|   IBIS model for TI xxx DSP
[IBIS Ver]   5.1
[Disclaimer]   Please be aware that in the absence of a written agreement
|   Texas Instruments(TI) assumes no liability for:
|   (1) The accuracy of the IBIS models provided to your company,
|   however, the IBIS model is compliant to industry standard
|   IQ Level 2a.  Refer to IBIS Quality Section below for
|   for full details.
|   (2) The proper functioning of these Models in your design
|   or for any resulting applications
|   (3) Infringement of patents, copyrights or intellectual
|   property rights resulting from your use of these
|   models.
|   TI provides IBIS Models as a service to our customers and
|   therefore reserves the right to limit distribution of the
|   Models.  The information is subject to change without notice.
[File Name]  sprm806c.ibs
[File Rev]   0.4
|   -Initial version
|   - Fixed component name
|   - Removed unsupported drive strengths for LVCMOS and SDIO models
|   - Removed unsupported drive strengths for LVDS, IIC and eMMC buffer models
[Date]   20 Oct 2023
[Source]   Texas Instruments Incorporated
[Copyright]   Property of Texas Instruments Incorporated.
|   Unauthorized reproduction and/or distribution is strictly.
|   prohibited.
|   This product is protected under copyright law and trade
|   secret law as an unpublished work.
|   Created 2012,(C) Copyright 1999-2012,
|   Texas Instruments Incorporated., All Rights Reserved.
|   These commodities are under the U.S. Government
|   distribution license control. As such,they are not to be
|   re-exported without the prior approval of the U.S.
|   Department of Commerce.
[Notes]
   This file does not include AMI models for SerDes based links.
   For SerDes simulations use Texas Instruments IBIS AMI models
   Some IV curves contain Non monotonic data points.
|   Revision History
|   GERNERAL COMMENT: All IBIS Quality Notes below reflect latest release
|   and version of IBIS File
|   File passes ibischk5.1 and ibischk6 with 0 errors and 119 warnings
|   Component AM62_AMC
[Component] AM62_AMC
[Manufacturer] Texas Instruments
[Package]
|   typ   min   max
R_pkg   0.44151   0.03098   0.71376
L_pkg   3.146e-9   4.999e-10   4.933e-9
C_pkg   1.051e-12   3.256e-13   1.586e-12
[Package Model]   am62_amc_pkg
[Pin]	Signal_name	model_name
C3	ATEST0	NC
R6	ATEST1	NC
T13	CSI0_ATB_0_H	NC
T14	CSI0_ATB_1_H	NC
AA14	CSI0_RXCLKN	NC
AA13	CSI0_RXCLKP	NC
Y13	CSI0_RXN0	NC
V13	CSI0_RXN1	NC
U12	CSI0_RXN2	NC
W12	CSI0_RXN3	NC
Y12	CSI0_RXP0	NC
V12	CSI0_RXP1	NC
U11	CSI0_RXP2	NC
W11	CSI0_RXP3	NC
T11	CSI0_RXRCALIB	NC
F5	DDR0_A0	DDR_SE
G5	DDR0_A1	DDR_SE
G4	DDR0_A2	DDR_SE
H4	DDR0_A3	DDR_SE
J5	DDR0_A4	DDR_SE
H5	DDR0_A5	DDR_SE
P4	DDR0_A6	DDR_SE
N2	DDR0_A7	DDR_SE
P2	DDR0_A8	DDR_SE
N4	DDR0_A9	DDR_SE
N3	DDR0_A10	DDR_SE
M3	DDR0_A11	DDR_SE
P5	DDR0_A12	DDR_SE
N5	DDR0_A13	DDR_SE
M1	DDR0_ACT_N	DDR_SE
N1	DDR0_ALERT_N	DDR_SE
M5	DDR0_ATB0	NC
M4	DDR0_ATB1	NC
L5	DDR0_BA0	DDR_SE
L3	DDR0_BA1	DDR_SE
L4	DDR0_BG0	DDR_SE
L2	DDR0_BG1	DDR_SE
K4	DDR0_CAL0	DDR_SE
J3	DDR0_CAS_N	DDR_SE
J1	DDR0_CK0	DDR_DIFF
K1	DDR0_CK0_N	DDR_DIFF
G3	DDR0_CKE0	DDR_SE
H2	DDR0_CKE1	DDR_SE
H3	DDR0_CS0_N	DDR_SE
G1	DDR0_CS1_N	DDR_SE
E3	DDR0_DM0	DDR_SE
R4	DDR0_DM1	DDR_SE
C2	DDR0_DQ0	DDR_SE
E4	DDR0_DQ1	DDR_SE
D3	DDR0_DQ2	DDR_SE
E5	DDR0_DQ3	DDR_SE
D2	DDR0_DQ4	DDR_SE
F3	DDR0_DQ5	DDR_SE
F1	DDR0_DQ6	DDR_SE
F2	DDR0_DQ7	DDR_SE
R3	DDR0_DQ8	DDR_SE
R2	DDR0_DQ9	DDR_SE
T2	DDR0_DQ10	DDR_SE
U2	DDR0_DQ11	DDR_SE
U3	DDR0_DQ12	DDR_SE
U4	DDR0_DQ13	DDR_SE
T4	DDR0_DQ14	DDR_SE
T5	DDR0_DQ15	DDR_SE
D1	DDR0_DQS0	DDR_DIFF
E1	DDR0_DQS0_N	DDR_DIFF
T1	DDR0_DQS1	DDR_DIFF
R1	DDR0_DQS1_N	DDR_DIFF
J4	DDR0_ODT0	DDR_SE
K2	DDR0_ODT1	DDR_SE
M2	DDR0_PAR	DDR_SE
K5	DDR0_RAS_N	DDR_SE
G2	DDR0_RESET0_N	DDR_SE
J2	DDR0_WE_N	DDR_SE
D9	EMU0	LVCMOS_V
B10	EMU1	LVCMOS_V
B16	EXTINTN	IIC_V
C14	EXT_REFCLK1	LVCMOS_V
K19	GPMC0_AD0	LVCMOS_H
L19	GPMC0_AD1	LVCMOS_H
L20	GPMC0_AD2	LVCMOS_H
L21	GPMC0_AD3	LVCMOS_H
M21	GPMC0_AD4	LVCMOS_H
L17	GPMC0_AD5	LVCMOS_H
L18	GPMC0_AD6	LVCMOS_H
M20	GPMC0_AD7	LVCMOS_H
N20	GPMC0_AD8	LVCMOS_H
N21	GPMC0_AD9	LVCMOS_H
M17	GPMC0_AD10	LVCMOS_H
N18	GPMC0_AD11	LVCMOS_H
N17	GPMC0_AD12	LVCMOS_H
N19	GPMC0_AD13	LVCMOS_H
P19	GPMC0_AD14	LVCMOS_H
P20	GPMC0_AD15	LVCMOS_H
K20	GPMC0_ADVN_ALE	LVCMOS_H
K17	GPMC0_BE0N_CLE	LVCMOS_H
K18	GPMC0_BE1N	LVCMOS_H
M19	GPMC0_CLK	LVCMOS_H
J18	GPMC0_CSN0	LVCMOS_H
H17	GPMC0_CSN1	LVCMOS_H
H18	GPMC0_CSN2	LVCMOS_H
H19	GPMC0_CSN3	LVCMOS_H
J19	GPMC0_DIR	LVCMOS_H
K21	GPMC0_OEN_REN	LVCMOS_H
P21	GPMC0_WAIT0	LVCMOS_H
P17	GPMC0_WAIT1	LVCMOS_H
J17	GPMC0_WEN	LVCMOS_H
J20	GPMC0_WPN	LVCMOS_H
E12	I2C0_SCL	LVCMOS_V
D14	I2C0_SDA	LVCMOS_V
A17	I2C1_SCL	LVCMOS_V
A16	I2C1_SDA	LVCMOS_V
E6	IFORCE	NC
A15	MCAN0_RX	LVCMOS_V
B13	MCAN0_TX	LVCMOS_V
D16	MCASP0_ACLKR	LVCMOS_V
C17	MCASP0_ACLKX	LVCMOS_V
D15	MCASP0_AFSR	LVCMOS_V
C16	MCASP0_AFSX	LVCMOS_V
D18	MCASP0_AXR0	LVCMOS_V
A18	MCASP0_AXR1	LVCMOS_V
B17	MCASP0_AXR2	LVCMOS_V
B18	MCASP0_AXR3	LVCMOS_V
B1	MCU_ERRORN	LVCMOS_H
B9	MCU_I2C0_SCL	IIC_V
A10	MCU_I2C0_SDA	IIC_V
C4	MCU_MCAN0_RX	LVCMOS_V
C5	MCU_MCAN0_TX	LVCMOS_V
D6	MCU_MCAN1_RX	LVCMOS_V
D5	MCU_MCAN1_TX	LVCMOS_V
A5	MCU_OSC0_XI	NC
A6	MCU_OSC0_XO	NC
B2	MCU_PORZ	RESET_H
A12	MCU_RESETSTATZ	LVCMOS_V
C9	MCU_RESETZ	LVCMOS_V
B7	MCU_SPI0_CLK	LVCMOS_V
E7	MCU_SPI0_CS0	LVCMOS_V
C8	MCU_SPI0_CS1	LVCMOS_V
E8	MCU_SPI0_D0	LVCMOS_V
D8	MCU_SPI0_D1	LVCMOS_V
B8	MCU_UART0_CTSN	LVCMOS_V
D7	MCU_UART0_RTSN	LVCMOS_V
A8	MCU_UART0_RXD	LVCMOS_V
B6	MCU_UART0_TXD	LVCMOS_V
V17	MDIO0_MDC	LVCMOS_V
U16	MDIO0_MDIO	LVCMOS_V
Y1	MMC0_CLK	SDIO_H
V3	MMC0_CMD	SDIO_H
V2	MMC0_DAT0	SDIO_H
V1	MMC0_DAT1	SDIO_H
W2	MMC0_DAT2	SDIO_H
W1	MMC0_DAT3	SDIO_H
Y2	MMC0_DAT4	SDIO_H
W3	MMC0_DAT5	SDIO_H
W4	MMC0_DAT6	SDIO_H
V4	MMC0_DAT7	SDIO_H
A20	MMC1_CLK	SDIO_V
C18	MMC1_CMD	SDIO_V
A19	MMC1_DAT0	SDIO_V
B19	MMC1_DAT1	SDIO_V
B20	MMC1_DAT2	SDIO_V
C19	MMC1_DAT3	SDIO_V
C15	MMC1_SDCD	LVCMOS_V
B15	MMC1_SDWP	LVCMOS_V
E21	MMC2_CLK	SDIO_H
C21	MMC2_CMD	SDIO_H
B21	MMC2_DAT0	SDIO_H
D21	MMC2_DAT1	SDIO_H
E19	MMC2_DAT2	SDIO_H
E20	MMC2_DAT3	SDIO_H
D20	MMC2_SDCD	LVCMOS_H
C20	MMC2_SDWP	LVCMOS_H
AA2	OLDI0_A0N	LVDS
AA3	OLDI0_A0P	LVDS
V5	OLDI0_A1N	LVDS
V6	OLDI0_A1P	LVDS
U7	OLDI0_A2N	LVDS
U6	OLDI0_A2P	LVDS
W6	OLDI0_A3N	LVDS
W5	OLDI0_A3P	LVDS
AA4	OLDI0_A4N	LVDS
Y5	OLDI0_A4P	LVDS
AA6	OLDI0_A5N	LVDS
AA5	OLDI0_A5P	LVDS
AA10	OLDI0_A6N	LVDS
Y9	OLDI0_A6P	LVDS
AA8	OLDI0_A7N	LVDS
Y8	OLDI0_A7P	LVDS
V7	OLDI0_CLK0N	LVDS
V8	OLDI0_CLK0P	LVDS
Y7	OLDI0_CLK1N	LVDS
AA7	OLDI0_CLK1P	LVDS
G19	OSPI0_CLK	LVCMOS_H
F19	OSPI0_CSN0	LVCMOS_H
F17	OSPI0_CSN1	LVCMOS_H
E17	OSPI0_CSN2	LVCMOS_H
E18	OSPI0_CSN3	LVCMOS_H
F18	OSPI0_D0	LVCMOS_H
G17	OSPI0_D1	LVCMOS_H
F21	OSPI0_D2	LVCMOS_H
F20	OSPI0_D3	LVCMOS_H
G21	OSPI0_D4	LVCMOS_H
H21	OSPI0_D5	LVCMOS_H
G20	OSPI0_D6	LVCMOS_H
J21	OSPI0_D7	LVCMOS_H
H20	OSPI0_DQS	LVCMOS_H
G18	OSPI0_LBCLKO	LVCMOS_H
C7	PMIC_LPM_EN0	LVCMOS_V
E13	PORZ_OUT	LVCMOS_V
E14	RESETSTATZ	LVCMOS_V
E15	RESET_REQZ	LVCMOS_V
W15	RGMII1_RD0	LVCMOS_V
Y16	RGMII1_RD1	LVCMOS_V
AA17	RGMII1_RD2	LVCMOS_V
Y15	RGMII1_RD3	LVCMOS_V
AA16	RGMII1_RXC	LVCMOS_V
W14	RGMII1_RX_CTL	LVCMOS_V
U14	RGMII1_TD0	LVCMOS_V
AA19	RGMII1_TD1	LVCMOS_V
Y17	RGMII1_TD2	LVCMOS_V
AA18	RGMII1_TD3	LVCMOS_V
W16	RGMII1_TXC	LVCMOS_V
V15	RGMII1_TX_CTL	LVCMOS_V
W18	RGMII2_RD0	LVCMOS_V
Y20	RGMII2_RD1	LVCMOS_V
Y19	RGMII2_RD2	LVCMOS_V
W20	RGMII2_RD3	LVCMOS_V
V18	RGMII2_RXC	LVCMOS_V
W19	RGMII2_RX_CTL	LVCMOS_V
AA20	RGMII2_TD0	LVCMOS_V
U15	RGMII2_TD1	LVCMOS_V
W17	RGMII2_TD2	LVCMOS_V
V16	RGMII2_TD3	LVCMOS_V
Y18	RGMII2_TXC	LVCMOS_V
Y21	RGMII2_TX_CTL	LVCMOS_V
D12	SPI0_CLK	LVCMOS_V
C11	SPI0_CS0	LVCMOS_V
D13	SPI0_CS1	LVCMOS_V
C12	SPI0_D0	LVCMOS_V
A14	SPI0_D1	LVCMOS_V
C10	TCK	LVCMOS_V
D10	TDI	LVCMOS_V
E10	TDO	LVCMOS_V
F8	TEMP_DIODE_P	NC
B11	TMS	LVCMOS_V
A11	TRSTN	LVCMOS_V
B14	UART0_CTSN	LVCMOS_V
C13	UART0_RTSN	LVCMOS_V
A13	UART0_RXD	LVCMOS_V
E11	UART0_TXD	LVCMOS_V
AA11	USB0_DM	NC
Y10	USB0_DP	NC
D17	USB0_DRVVBUS	LVCMOS_V
T8	USB0_RCALIB	NC
V10	USB0_VBUS	NC
W8	USB1_DM	NC
W9	USB1_DP	NC
E16	USB1_DRVVBUS	LVCMOS_V
V9	USB1_RCALIB	NC
U9	USB1_VBUS	NC
J7	VDDS_OSC0	POWER
H9	VMON_1P8_SOC	POWER
K11	VMON_3P3_SOC	POWER
F6	VMON_ER_VSYS	POWER
R21	VOUT0_DATA0	LVCMOS_H
P18	VOUT0_DATA1	LVCMOS_H
R18	VOUT0_DATA2	LVCMOS_H
R19	VOUT0_DATA3	LVCMOS_H
R20	VOUT0_DATA4	LVCMOS_H
T20	VOUT0_DATA5	LVCMOS_H
T21	VOUT0_DATA6	LVCMOS_H
T19	VOUT0_DATA7	LVCMOS_H
U21	VOUT0_DATA8	LVCMOS_H
R17	VOUT0_DATA9	LVCMOS_H
T18	VOUT0_DATA10	LVCMOS_H
U20	VOUT0_DATA11	LVCMOS_H
U19	VOUT0_DATA12	LVCMOS_H
V21	VOUT0_DATA13	LVCMOS_H
U18	VOUT0_DATA14	LVCMOS_H
V20	VOUT0_DATA15	LVCMOS_H
T17	VOUT0_DE	LVCMOS_H
W21	VOUT0_HSYNC	LVCMOS_H
U17	VOUT0_PCLK	LVCMOS_H
T16	VOUT0_VSYNC	LVCMOS_H
B3	VSENSE	NC
B12	WKUP_CLKOUT0	LVCMOS_V
E9	WKUP_I2C0_SCL	IIC_V
A9	WKUP_I2C0_SDA	IIC_V
A2	WKUP_LFOSC0_XI	NC
A3	WKUP_LFOSC0_XO	NC
A7	WKUP_UART0_CTSN	LVCMOS_V
B4	WKUP_UART0_RTSN	LVCMOS_V
B5	WKUP_UART0_RXD	LVCMOS_V
C6	WKUP_UART0_TXD	LVCMOS_V
Y6	VSS	GND
Y4	VSS	GND
Y3	VSS	GND
Y14	VSS	GND
Y11	VSS	GND
W7	VSS	GND
W13	VSS	GND
W10	VSS	GND
V19	VSS	GND
V14	VSS	GND
V11	VSS	GND
U8	VSS	GND
U5	VSS	GND
U13	VSS	GND
U10	VSS	GND
T9	VSS	GND
T7	VSS	GND
T6	VSS	GND
T3	VSS	GND
T15	VSS	GND
T12	VSS	GND
T10	VSS	GND
R8	VSS	GND
R7	VSS	GND
R5	VSS	GND
R16	VSS	GND
P6	VSS	GND
P3	VSS	GND
P16	VSS	GND
P15	VSS	GND
P13	VSS	GND
P10	VSS	GND
P1	VSS	GND
N6	VSS	GND
N14	VSS	GND
N12	VSS	GND
M9	VSS	GND
M6	VSS	GND
M18	VSS	GND
M16	VSS	GND
M11	VSS	GND
L6	VSS	GND
L16	VSS	GND
L14	VSS	GND
L10	VSS	GND
L1	VSS	GND
K8	VSS	GND
K6	VSS	GND
K3	VSS	GND
K13	VSS	GND
J6	VSS	GND
J16	VSS	GND
J14	VSS	GND
J12	VSS	GND
J10	VSS	GND
H6	VSS	GND
H13	VSS	GND
H1	VSS	GND
G9	VSS	GND
G6	VSS	GND
G16	VSS	GND
F9	VSS	GND
F4	VSS	GND
F15	VSS	GND
F13	VSS	GND
F11	VSS	GND
E2	VSS	GND
D4	VSS	GND
D19	VSS	GND
D11	VSS	GND
AA9	VSS	GND
AA21	VSS	GND
AA15	VSS	GND
AA12	VSS	GND
AA1	VSS	GND
A4	VSS	GND
A21	VSS	GND
A1	VSS	GND
L12	VSS	GND
G12	CAP_VDDS0	POWER
L15	CAP_VDDS1	POWER
R13	CAP_VDDS2	POWER
M15	CAP_VDDS3	POWER
N8	CAP_VDDS4	POWER
G15	CAP_VDDS5	POWER
J15	CAP_VDDS6	POWER
G8	CAP_VDDS_CANUART	POWER
G11	CAP_VDDS_MCU	POWER
R12	VDDA_1P8_CSIRX0	POWER
R9	VDDA_1P8_OLDI0	POWER
P9	VDDA_1P8_OLDI0	POWER
R11	VDDA_1P8_USB	POWER
R10	VDDA_3P3_USB	POWER
P12	VDDA_CORE_CSIRX0	POWER
P11	VDDA_CORE_USB	POWER
L9	VDDA_DDR_PLL0	POWER
H10	VDDA_MCU	POWER
N10	VDDA_PLL0	POWER
P14	VDDA_PLL1	POWER
K12	VDDA_PLL2	POWER
M7	VDDA_TEMP0	POWER
F16	VDDA_TEMP1	POWER
M13	VDDR_CORE	POWER
H11	VDDR_CORE	POWER
M10	VDDR_CORE	POWER
G13	VDDSHV0	POWER
F12	VDDSHV0	POWER
K16	VDDSHV1	POWER
K15	VDDSHV1	POWER
R15	VDDSHV2	POWER
R14	VDDSHV2	POWER
N16	VDDSHV3	POWER
N15	VDDSHV3	POWER
P7	VDDSHV4	POWER
N7	VDDSHV4	POWER
G14	VDDSHV5	POWER
F14	VDDSHV5	POWER
H16	VDDSHV6	POWER
H15	VDDSHV6	POWER
H7	VDDSHV_CANUART	POWER
G7	VDDSHV_CANUART	POWER
G10	VDDSHV_MCU	POWER
F10	VDDSHV_MCU	POWER
C1	VDDS_DDR	POWER
J8	VDDS_DDR	POWER
K7	VDDS_DDR	POWER
K9	VDDS_DDR	POWER
L8	VDDS_DDR	POWER
U1	VDDS_DDR	POWER
L7	VDDS_DDR_C	POWER
H8	VDD_CANUART	POWER
P8	VDD_CORE	POWER
N9	VDD_CORE	POWER
N13	VDD_CORE	POWER
N11	VDD_CORE	POWER
M8	VDD_CORE	POWER
M14	VDD_CORE	POWER
M12	VDD_CORE	POWER
L13	VDD_CORE	POWER
L11	VDD_CORE	POWER
K14	VDD_CORE	POWER
K10	VDD_CORE	POWER
J9	VDD_CORE	POWER
J13	VDD_CORE	POWER
J11	VDD_CORE	POWER
H14	VDD_CORE	POWER
H12	VDD_CORE	POWER
F7	VPP	POWER
|********************  DIFF PIN  *******************************
[Diff_pin]   inv_pin vdiff tdelay_typ   tdelay_min  tdelay_max
J1	K1	NA	NA	NA	NA	||	DDR0_CK0	&	DDR0_CK0_N
D1	E1	NA	NA	NA	NA	||	DDR0_DQS0	&	DDR0_DQS0_N
T1	R1	NA	NA	NA	NA	||	DDR0_DQS1	&	DDR0_DQS1_N
AA2	AA3	NA	NA	NA	NA	||	OLDI0_A0N	&	OLDI0_A0P
V5	V6	NA	NA	NA	NA	||	OLDI0_A1N	&	OLDI0_A1P
U7	U6	NA	NA	NA	NA	||	OLDI0_A2N	&	OLDI0_A2P
W6	W5	NA	NA	NA	NA	||	OLDI0_A3N	&	OLDI0_A3P
AA4	Y5	NA	NA	NA	NA	||	OLDI0_A4N	&	OLDI0_A4P
AA6	AA5	NA	NA	NA	NA	||	OLDI0_A5N	&	OLDI0_A5P
AA10	Y9	NA	NA	NA	NA	||	OLDI0_A6N	&	OLDI0_A6P
AA8	Y8	NA	NA	NA	NA	||	OLDI0_A7N	&	OLDI0_A7P
V7	V8	NA	NA	NA	NA	||	OLDI0_CLK0N	&	OLDI0_CLK0P
Y7	AA7	NA	NA	NA	NA	||	OLDI0_CLK1N	&	OLDI0_CLK1P
|---------------- DDR -------------------
[Model Selector] DDR_SE
lpddr4_ocd_240p_240n  driver with 240 ohms pullup and 240 ohms pulldown strength
lpddr4_ocd_120p_120n  driver with 120 ohms pullup and 120 ohms pulldown strength
lpddr4_ocd_80p_80n  driver with 80 ohms pullup and 80 ohms pulldown strength
lpddr4_ocd_60p_60n  driver with 60 ohms pullup and 60 ohms pulldown strength
lpddr4_ocd_48p_48n  driver with 48 ohms pullup and 48 ohms pulldown strength
lpddr4_ocd_40p_40n  driver with 40 ohms pullup and 40 ohms pulldown strength
lpddr4_ocd_120pd_60p_40n  driver with 60/40 ohms pullup/pulldown 120 ohms aopd strength
lpddr4_ocd_120pd_48p_40n  driver with 48/40 ohms pullup/pulldown 120 ohms aopd strength
lp4x_ocd_34p_34n  driver with 34 ohms pullup and 34 ohms pulldown strength
lp4x_ocd_40p_40n  driver with 40 ohms pullup and 40 ohms pulldown strength
lp4x_ocd_48p_48n  driver with 48 ohms pullup and 48 ohms pulldown strength
lp4x_ocd_60p_60n  driver with 60 ohms pullup and 60 ohms pulldown strength
lp4x_ocd_80p_80n  driver with 80 ohms pullup and 80 ohms pulldown strength
lp4x_ocd_120p_120n  driver with 120 ohms pullup and 120 ohms pulldown strength
lp4x_ocd_240p_240n  driver with 240 ohms pullup and 240 ohms pulldown strength
lp4x_0p6_ocd_80p_80n  driver with 80 ohms pullup and 80 ohms pulldown strength
lp4x_0p6_ocd_40p_40n  driver with 40 ohms pullup and 40 ohms pulldown strength
lpddr4_odt_240  240 ohm termination
lpddr4_odt_120  120 ohm termination
lpddr4_odt_80  80 ohm termination
lpddr4_odt_60  60 ohm termination
lpddr4_odt_48  48 ohm termination
lpddr4_odt_40  40 ohm termination
lpddr4_odt_off  open ohm termination
lp4x_odt_40  40 ohm termination
lp4x_odt_48  48 ohm termination
lp4x_odt_60  60 ohm termination
lp4x_odt_80  80 ohm termination
lp4x_odt_120  120 ohm termination
lp4x_odt_240  240 ohm termination
lp4x_odt_off  open
ddr4_ocd_34p_34n  driver with 34 ohms pullup and 34 ohms pulldown strength, max slew rate
ddr4_ocd_40p_40n  driver with 40 ohms pullup and 40 ohms pulldown strength, max slew rate
ddr4_ocd_48p_48n  driver with 48 ohms pullup and 48 ohms pulldown strength, max slew rate
ddr4_ocd_60p_60n  driver with 60 ohms pullup and 60 ohms pulldown strength, max slew rate
ddr4_ocd_80p_80n  driver with 80 ohms pullup and 80 ohms pulldown strength, max slew rate
ddr4_odt_34  34 ohm termination
ddr4_odt_40  40 ohm termination
ddr4_odt_48  48 ohm termination
ddr4_odt_60  60 ohm termination
ddr4_odt_80  80 ohm termination
ddr4_odt_120  120 ohm termination
ddr4_odt_240  240 ohm termination
ddr4_odt_off  No termination
[Model Selector] DDR_DIFF
lpddr4_ocd_240p_240n_diff  driver with 240 ohms pullup and 240 ohms pulldown strength
lpddr4_ocd_120p_120n_diff  driver with 120 ohms pullup and 120 ohms pulldown strength
lpddr4_ocd_80p_80n_diff  driver with 80 ohms pullup and 80 ohms pulldown strength
lpddr4_ocd_60p_60n_diff  driver with 60 ohms pullup and 60 ohms pulldown strength
lpddr4_ocd_48p_48n_diff  driver with 48 ohms pullup and 48 ohms pulldown strength
lpddr4_ocd_40p_40n_diff  driver with 40 ohms pullup and 40 ohms pulldown strength
lpddr4_ocd_120pd_60p_40n_diff  driver with 60/40 ohms pullup/pulldown 120 ohms aopd strength
lpddr4_ocd_120pd_48p_40n_diff  driver with 48/40 ohms pullup/pulldown 120 ohms aopd strength
lp4x_ocd_34p_34n_diff  driver with 34 ohms pullup and 34 ohms pulldown strength
lp4x_ocd_40p_40n_diff  driver with 40 ohms pullup and 40 ohms pulldown strength
lp4x_ocd_48p_48n_diff  driver with 48 ohms pullup and 48 ohms pulldown strength
lp4x_ocd_60p_60n_diff  driver with 60 ohms pullup and 60 ohms pulldown strength
lp4x_ocd_80p_80n_diff  driver with 80 ohms pullup and 80 ohms pulldown strength
lp4x_ocd_120p_120n_diff  driver with 120 ohms pullup and 120 ohms pulldown strength
lp4x_ocd_240p_240n_diff  driver with 240 ohms pullup and 240 ohms pulldown strength
lp4x_0p6_ocd_80p_80n_diff  driver with 80 ohms pullup and 80 ohms pulldown strength
lp4x_0p6_ocd_40p_40n_diff  driver with 40 ohms pullup and 40 ohms pulldown strength
lpddr4_odt_240_diff  240 ohm termination
lpddr4_odt_120_diff  120 ohm termination
lpddr4_odt_80_diff  80 ohm termination
lpddr4_odt_60_diff  60 ohm termination
lpddr4_odt_48_diff  48 ohm termination
lpddr4_odt_40_diff  40 ohm termination
lpddr4_odt_off_diff  open ohm termination
lp4x_odt_40_diff  40 ohm termination
lp4x_odt_48_diff  48 ohm termination
lp4x_odt_60_diff  60 ohm termination
lp4x_odt_80_diff  80 ohm termination
lp4x_odt_120_diff  120 ohm termination
lp4x_odt_240_diff  240 ohm termination
lp4x_odt_off_diff  open
ddr4_ocd_34p_34n_diff  driver with 34 ohms pullup and 34 ohms pulldown strength, max slew rate
ddr4_ocd_40p_40n_diff  driver with 40 ohms pullup and 40 ohms pulldown strength, max slew rate
ddr4_ocd_48p_48n_diff  driver with 48 ohms pullup and 48 ohms pulldown strength, max slew rate
ddr4_ocd_60p_60n_diff  driver with 60 ohms pullup and 60 ohms pulldown strength, max slew rate
ddr4_ocd_80p_80n_diff  driver with 80 ohms pullup and 80 ohms pulldown strength, max slew rate
ddr4_odt_34_diff  34 ohm termination
ddr4_odt_40_diff  40 ohm termination
ddr4_odt_48_diff  48 ohm termination
ddr4_odt_60_diff  60 ohm termination
ddr4_odt_80_diff  80 ohm termination
ddr4_odt_120_diff  120 ohm termination
ddr4_odt_240_diff  240 ohm termination
ddr4_odt_off_diff  No termination
|****************** SDIO
[Model Selector] SDIO_H
sdio1_r40_1p8_h PRWDWUWSWEWCDGSDIO_H@_R40_1p8_comment
sdio1_r40_3p3_h PRWDWUWSWEWCDGSDIO_H@_R40_3p3_comment
[Model Selector] SDIO_V
sdio0_r40_1p8_v PRWDWUWSWEWCDGSDIO_V@_R40_1p8_comment
sdio0_r40_3p3_v PRWDWUWSWEWCDGSDIO_V@_R40_3p3_comment
|********** LVCMOS
[Model Selector] LVCMOS_H
lvcmos1_nom_1p8_h PRWDWUWSWEWCDGLVCMOS_H@_Nom_1p8_comment
lvcmos1_nom_3p3_h PRWDWUWSWEWCDGLVCMOS_H@_Nom_3p3_comment
[Model Selector] LVCMOS_V
lvcmos0_nom_1p8_v PRWDWUWSWEWCDGLVCMOS_V@_Nom_1p8_comment
lvcmos0_nom_3p3_v PRWDWUWSWEWCDGLVCMOS_V@_Nom_3p3_comment
[Model Selector] IIC_V
IIC18_1_0_V PRBOPDDGZIIC_V@HSMODE_HSMCSE=0_0_comment 1.8V
IIC18_1_1_V PRBOPDDGZIIC_V@HSMODE_HSMCSE=0_1_comment 1.8V
IIC18_1_2_V PRBOPDDGZIIC_V@HSMODE_HSMCSE=1_0_comment 1.8V
IIC18_1_3_V PRBOPDDGZIIC_V@HSMODE_HSMCSE=1_1_comment 1.8V
IIC33_1_0_V PRBOPDDGZIIC_V@HSMODE_HSMCSE=0_0_comment
[Model Selector] LVDS
lvds_tx_03   LVDS TX Driver Permumentation 03
lvds_tx_11   LVDS TX Driver Permumentation 11
|***************** RESET ************************************************
[Model Selector] RESET_H
reset18_0_0 PDIDGZRESET_H
|   EMMC
[MODEL SELECTOR] EMMC
emmc51_io_tx40ohm   40ohm DRIVER
|   Package Model
[Define Package Model]   am62_amc_pkg
[Manufacturer]   name 1
[OEM]   name 2
[Description]   330-pin Package
|[Number of Sections]   1
[Number of Pins]   330
[Pin Numbers]
|[Pin Name]  Net Number   Net Name   Net's All Pins
G12   | 1   CAP_VDDS0   G12
L15   | 2   CAP_VDDS1   L15
R13   | 3   CAP_VDDS2   R13
M15   | 4   CAP_VDDS3   M15
N8   | 5   CAP_VDDS4   N8
G15   | 6   CAP_VDDS5   G15
J15   | 7   CAP_VDDS6   J15
G8   | 8   CAP_VDDS_CANUART   G8
G11   | 9   CAP_VDDS_MCU   G11
R12   | 10   VDDA_1P8_CSIRX0   R12
R9   | 11   VDDA_1P8_OLDI0   R9
   |P9
R11   | 12   VDDA_1P8_USB   R11
R10   | 13   VDDA_3P3_USB   R10
P12   | 14   VDDA_CORE_CSIRX0   P12
P11   | 15   VDDA_CORE_USB   P11
L9   | 16   VDDA_DDR_PLL0   L9
H10   | 17   VDDA_MCU   H10
N10   | 18   VDDA_PLL0   N10
P14   | 19   VDDA_PLL1   P14
K12   | 20   VDDA_PLL2   K12
M7   | 21   VDDA_TEMP0   M7
F16   | 22   VDDA_TEMP1   F16
M13   | 23   VDDR_CORE   M13
   |H11
   |M10
G13   | 24   VDDSHV0   G13
   |F12
K16   | 25   VDDSHV1   K16
   |K15
R15   | 26   VDDSHV2   R15
   |R14
N16   | 27   VDDSHV3   N16
   |N15
P7   | 28   VDDSHV4   P7
   |N7
G14   | 29   VDDSHV5   G14
   |F14
H16   | 30   VDDSHV6   H16
   |H15
H7   | 31   VDDSHV_CANUART   H7
   |G7
G10   | 32   VDDSHV_MCU   G10
   |F10
C1   | 33   VDDS_DDR   C1
   |J8
   |K7
   |K9
   |L8
   |U1
L7   | 34   VDDS_DDR_C   L7
H8   | 35   VDD_CANUART   H8
P8   | 36   VDD_CORE   P8
   |N9
   |N13
   |N11
   |M8
   |M14
   |M12
   |L13
   |L11
   |K14
   |K10
   |J9
   |J13
   |J11
   |H14
   |H12
F7   | 37   VPP   F7
C3   | 38   ATEST0   C3
R6   | 39   ATEST1   R6
T13   | 40   CSI0_ATB_0_H   T13
T14   | 41   CSI0_ATB_1_H   T14
AA14   | 42   CSI0_RXCLKN   AA14
AA13   | 43   CSI0_RXCLKP   AA13
Y13   | 44   CSI0_RXN0   Y13
V13   | 45   CSI0_RXN1   V13
U12   | 46   CSI0_RXN2   U12
W12   | 47   CSI0_RXN3   W12
Y12   | 48   CSI0_RXP0   Y12
V12   | 49   CSI0_RXP1   V12
U11   | 50   CSI0_RXP2   U11
W11   | 51   CSI0_RXP3   W11
T11   | 52   CSI0_RXRCALIB   T11
F5   | 53   DDR0_A0   F5
G5   | 54   DDR0_A1   G5
G4   | 55   DDR0_A2   G4
H4   | 56   DDR0_A3   H4
J5   | 57   DDR0_A4   J5
H5   | 58   DDR0_A5   H5
P4   | 59   DDR0_A6   P4
N2   | 60   DDR0_A7   N2
P2   | 61   DDR0_A8   P2
N4   | 62   DDR0_A9   N4
N3   | 63   DDR0_A10   N3
M3   | 64   DDR0_A11   M3
P5   | 65   DDR0_A12   P5
N5   | 66   DDR0_A13   N5
M1   | 67   DDR0_ACT_N   M1
N1   | 68   DDR0_ALERT_N   N1
M5   | 69   DDR0_ATB0   M5
M4   | 70   DDR0_ATB1   M4
L5   | 71   DDR0_BA0   L5
L3   | 72   DDR0_BA1   L3
L4   | 73   DDR0_BG0   L4
L2   | 74   DDR0_BG1   L2
K4   | 75   DDR0_CAL0   K4
J3   | 76   DDR0_CAS_N   J3
J1   | 77   DDR0_CK0   J1
K1   | 78   DDR0_CK0_N   K1
G3   | 79   DDR0_CKE0   G3
H2   | 80   DDR0_CKE1   H2
H3   | 81   DDR0_CS0_N   H3
G1   | 82   DDR0_CS1_N   G1
E3   | 83   DDR0_DM0   E3
R4   | 84   DDR0_DM1   R4
C2   | 85   DDR0_DQ0   C2
E4   | 86   DDR0_DQ1   E4
D3   | 87   DDR0_DQ2   D3
E5   | 88   DDR0_DQ3   E5
D2   | 89   DDR0_DQ4   D2
F3   | 90   DDR0_DQ5   F3
F1   | 91   DDR0_DQ6   F1
F2   | 92   DDR0_DQ7   F2
R3   | 93   DDR0_DQ8   R3
R2   | 94   DDR0_DQ9   R2
T2   | 95   DDR0_DQ10   T2
U2   | 96   DDR0_DQ11   U2
U3   | 97   DDR0_DQ12   U3
U4   | 98   DDR0_DQ13   U4
T4   | 99   DDR0_DQ14   T4
T5   | 100   DDR0_DQ15   T5
D1   | 101   DDR0_DQS0   D1
E1   | 102   DDR0_DQS0_N   E1
T1   | 103   DDR0_DQS1   T1
R1   | 104   DDR0_DQS1_N   R1
J4   | 105   DDR0_ODT0   J4
K2   | 106   DDR0_ODT1   K2
M2   | 107   DDR0_PAR   M2
K5   | 108   DDR0_RAS_N   K5
G2   | 109   DDR0_RESET0_N   G2
J2   | 110   DDR0_WE_N   J2
D9   | 111   EMU0   D9
B10   | 112   EMU1   B10
B16   | 113   EXTINTN   B16
C14   | 114   EXT_REFCLK1   C14
K19   | 115   GPMC0_AD0   K19
L19   | 116   GPMC0_AD1   L19
L20   | 117   GPMC0_AD2   L20
L21   | 118   GPMC0_AD3   L21
M21   | 119   GPMC0_AD4   M21
L17   | 120   GPMC0_AD5   L17
L18   | 121   GPMC0_AD6   L18
M20   | 122   GPMC0_AD7   M20
N20   | 123   GPMC0_AD8   N20
N21   | 124   GPMC0_AD9   N21
M17   | 125   GPMC0_AD10   M17
N18   | 126   GPMC0_AD11   N18
N17   | 127   GPMC0_AD12   N17
N19   | 128   GPMC0_AD13   N19
P19   | 129   GPMC0_AD14   P19
P20   | 130   GPMC0_AD15   P20
K20   | 131   GPMC0_ADVN_ALE   K20
K17   | 132   GPMC0_BE0N_CLE   K17
K18   | 133   GPMC0_BE1N   K18
M19   | 134   GPMC0_CLK   M19
J18   | 135   GPMC0_CSN0   J18
H17   | 136   GPMC0_CSN1   H17
H18   | 137   GPMC0_CSN2   H18
H19   | 138   GPMC0_CSN3   H19
J19   | 139   GPMC0_DIR   J19
K21   | 140   GPMC0_OEN_REN   K21
P21   | 141   GPMC0_WAIT0   P21
P17   | 142   GPMC0_WAIT1   P17
J17   | 143   GPMC0_WEN   J17
J20   | 144   GPMC0_WPN   J20
E12   | 145   I2C0_SCL   E12
D14   | 146   I2C0_SDA   D14
A17   | 147   I2C1_SCL   A17
A16   | 148   I2C1_SDA   A16
E6   | 149   IFORCE   E6
A15   | 150   MCAN0_RX   A15
B13   | 151   MCAN0_TX   B13
D16   | 152   MCASP0_ACLKR   D16
C17   | 153   MCASP0_ACLKX   C17
D15   | 154   MCASP0_AFSR   D15
C16   | 155   MCASP0_AFSX   C16
D18   | 156   MCASP0_AXR0   D18
A18   | 157   MCASP0_AXR1   A18
B17   | 158   MCASP0_AXR2   B17
B18   | 159   MCASP0_AXR3   B18
B1   | 160   MCU_ERRORN   B1
B9   | 161   MCU_I2C0_SCL   B9
A10   | 162   MCU_I2C0_SDA   A10
C4   | 163   MCU_MCAN0_RX   C4
C5   | 164   MCU_MCAN0_TX   C5
D6   | 165   MCU_MCAN1_RX   D6
D5   | 166   MCU_MCAN1_TX   D5
A5   | 167   MCU_OSC0_XI   A5
A6   | 168   MCU_OSC0_XO   A6
B2   | 169   MCU_PORZ   B2
A12   | 170   MCU_RESETSTATZ   A12
C9   | 171   MCU_RESETZ   C9
B7   | 172   MCU_SPI0_CLK   B7
E7   | 173   MCU_SPI0_CS0   E7
C8   | 174   MCU_SPI0_CS1   C8
E8   | 175   MCU_SPI0_D0   E8
D8   | 176   MCU_SPI0_D1   D8
B8   | 177   MCU_UART0_CTSN   B8
D7   | 178   MCU_UART0_RTSN   D7
A8   | 179   MCU_UART0_RXD   A8
B6   | 180   MCU_UART0_TXD   B6
V17   | 181   MDIO0_MDC   V17
U16   | 182   MDIO0_MDIO   U16
Y1   | 183   MMC0_CLK   Y1
V3   | 184   MMC0_CMD   V3
V2   | 185   MMC0_DAT0   V2
V1   | 186   MMC0_DAT1   V1
W2   | 187   MMC0_DAT2   W2
W1   | 188   MMC0_DAT3   W1
Y2   | 189   MMC0_DAT4   Y2
W3   | 190   MMC0_DAT5   W3
W4   | 191   MMC0_DAT6   W4
V4   | 192   MMC0_DAT7   V4
A20   | 193   MMC1_CLK   A20
C18   | 194   MMC1_CMD   C18
A19   | 195   MMC1_DAT0   A19
B19   | 196   MMC1_DAT1   B19
B20   | 197   MMC1_DAT2   B20
C19   | 198   MMC1_DAT3   C19
C15   | 199   MMC1_SDCD   C15
B15   | 200   MMC1_SDWP   B15
E21   | 201   MMC2_CLK   E21
C21   | 202   MMC2_CMD   C21
B21   | 203   MMC2_DAT0   B21
D21   | 204   MMC2_DAT1   D21
E19   | 205   MMC2_DAT2   E19
E20   | 206   MMC2_DAT3   E20
D20   | 207   MMC2_SDCD   D20
C20   | 208   MMC2_SDWP   C20
AA2   | 209   OLDI0_A0N   AA2
AA3   | 210   OLDI0_A0P   AA3
V5   | 211   OLDI0_A1N   V5
V6   | 212   OLDI0_A1P   V6
U7   | 213   OLDI0_A2N   U7
U6   | 214   OLDI0_A2P   U6
W6   | 215   OLDI0_A3N   W6
W5   | 216   OLDI0_A3P   W5
AA4   | 217   OLDI0_A4N   AA4
Y5   | 218   OLDI0_A4P   Y5
AA6   | 219   OLDI0_A5N   AA6
AA5   | 220   OLDI0_A5P   AA5
AA10   | 221   OLDI0_A6N   AA10
Y9   | 222   OLDI0_A6P   Y9
AA8   | 223   OLDI0_A7N   AA8
Y8   | 224   OLDI0_A7P   Y8
V7   | 225   OLDI0_CLK0N   V7
V8   | 226   OLDI0_CLK0P   V8
Y7   | 227   OLDI0_CLK1N   Y7
AA7   | 228   OLDI0_CLK1P   AA7
G19   | 229   OSPI0_CLK   G19
F19   | 230   OSPI0_CSN0   F19
F17   | 231   OSPI0_CSN1   F17
E17   | 232   OSPI0_CSN2   E17
E18   | 233   OSPI0_CSN3   E18
F18   | 234   OSPI0_D0   F18
G17   | 235   OSPI0_D1   G17
F21   | 236   OSPI0_D2   F21
F20   | 237   OSPI0_D3   F20
G21   | 238   OSPI0_D4   G21
H21   | 239   OSPI0_D5   H21
G20   | 240   OSPI0_D6   G20
J21   | 241   OSPI0_D7   J21
H20   | 242   OSPI0_DQS   H20
G18   | 243   OSPI0_LBCLKO   G18
C7   | 244   PMIC_LPM_EN0   C7
E13   | 245   PORZ_OUT   E13
E14   | 246   RESETSTATZ   E14
E15   | 247   RESET_REQZ   E15
W15   | 248   RGMII1_RD0   W15
Y16   | 249   RGMII1_RD1   Y16
AA17   | 250   RGMII1_RD2   AA17
Y15   | 251   RGMII1_RD3   Y15
AA16   | 252   RGMII1_RXC   AA16
W14   | 253   RGMII1_RX_CTL   W14
U14   | 254   RGMII1_TD0   U14
AA19   | 255   RGMII1_TD1   AA19
Y17   | 256   RGMII1_TD2   Y17
AA18   | 257   RGMII1_TD3   AA18
W16   | 258   RGMII1_TXC   W16
V15   | 259   RGMII1_TX_CTL   V15
W18   | 260   RGMII2_RD0   W18
Y20   | 261   RGMII2_RD1   Y20
Y19   | 262   RGMII2_RD2   Y19
W20   | 263   RGMII2_RD3   W20
V18   | 264   RGMII2_RXC   V18
W19   | 265   RGMII2_RX_CTL   W19
AA20   | 266   RGMII2_TD0   AA20
U15   | 267   RGMII2_TD1   U15
W17   | 268   RGMII2_TD2   W17
V16   | 269   RGMII2_TD3   V16
Y18   | 270   RGMII2_TXC   Y18
Y21   | 271   RGMII2_TX_CTL   Y21
D12   | 272   SPI0_CLK   D12
C11   | 273   SPI0_CS0   C11
D13   | 274   SPI0_CS1   D13
C12   | 275   SPI0_D0   C12
A14   | 276   SPI0_D1   A14
C10   | 277   TCK   C10
D10   | 278   TDI   D10
E10   | 279   TDO   E10
F8   | 280   TEMP_DIODE_P   F8
B11   | 281   TMS   B11
A11   | 282   TRSTN   A11
B14   | 283   UART0_CTSN   B14
C13   | 284   UART0_RTSN   C13
A13   | 285   UART0_RXD   A13
E11   | 286   UART0_TXD   E11
AA11   | 287   USB0_DM   AA11
Y10   | 288   USB0_DP   Y10
D17   | 289   USB0_DRVVBUS   D17
T8   | 290   USB0_RCALIB   T8
V10   | 291   USB0_VBUS   V10
W8   | 292   USB1_DM   W8
W9   | 293   USB1_DP   W9
E16   | 294   USB1_DRVVBUS   E16
V9   | 295   USB1_RCALIB   V9
U9   | 296   USB1_VBUS   U9
J7   | 297   VDDS_OSC0   J7
H9   | 298   VMON_1P8_SOC   H9
K11   | 299   VMON_3P3_SOC   K11
F6   | 300   VMON_ER_VSYS   F6
R21   | 301   VOUT0_DATA0   R21
P18   | 302   VOUT0_DATA1   P18
R18   | 303   VOUT0_DATA2   R18
R19   | 304   VOUT0_DATA3   R19
R20   | 305   VOUT0_DATA4   R20
T20   | 306   VOUT0_DATA5   T20
T21   | 307   VOUT0_DATA6   T21
T19   | 308   VOUT0_DATA7   T19
U21   | 309   VOUT0_DATA8   U21
R17   | 310   VOUT0_DATA9   R17
T18   | 311   VOUT0_DATA10   T18
U20   | 312   VOUT0_DATA11   U20
U19   | 313   VOUT0_DATA12   U19
V21   | 314   VOUT0_DATA13   V21
U18   | 315   VOUT0_DATA14   U18
V20   | 316   VOUT0_DATA15   V20
T17   | 317   VOUT0_DE   T17
W21   | 318   VOUT0_HSYNC   W21
U17   | 319   VOUT0_PCLK   U17
T16   | 320   VOUT0_VSYNC   T16
B3   | 321   VSENSE   B3
B12   | 322   WKUP_CLKOUT0   B12
E9   | 323   WKUP_I2C0_SCL   E9
A9   | 324   WKUP_I2C0_SDA   A9
A2   | 325   WKUP_LFOSC0_XI   A2
A3   | 326   WKUP_LFOSC0_XO   A3
A7   | 327   WKUP_UART0_CTSN   A7
B4   | 328   WKUP_UART0_RTSN   B4
B5   | 329   WKUP_UART0_RXD   B5
C6   | 330   WKUP_UART0_TXD   C6
[Model Data]
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[End Model Data]
[End Package Model]
| Models and submodels in the file (137): lvcmos1_nom_1p8_h (I/O), lvcmos0_nom_1p8_v (I/O), lvcmos1_nom_3p3_h (I/O), lvcmos0_nom_3p3_v (I/O), sdio1_r40_1p8_h (I/O), sdio0_r40_1p8_v (I/O), sdio1_r40_3p3_h (I/O), sdio0_r40_3p3_v (I/O), lpddr4_odt_120 (Input), lpddr4_odt_120_diff (Input), lpddr4_ocd_120p_120n (I/O), lpddr4_ocd_240p_240n (I/O), lpddr4_odt_240 (Input), lpddr4_ocd_40p_40n (I/O), lpddr4_odt_40 (Input), lpddr4_ocd_48p_48n (I/O), lpddr4_odt_48 (Input), lpddr4_ocd_60p_60n (I/O), lpddr4_odt_60 (Input), lpddr4_ocd_80p_80n (I/O), lpddr4_odt_80 (Input), lpddr4_odt_off (Input), lpddr4_ocd_120pd_60p_40n (I/O), lpddr4_ocd_120p_120n_diff (I/O), lpddr4_ocd_240p_240n_diff (I/O), lpddr4_odt_240_diff (Input), lpddr4_ocd_40p_40n_diff (I/O), lpddr4_odt_40_diff (Input), lpddr4_ocd_48p_48n_diff (I/O), lpddr4_odt_48_diff (Input), lpddr4_ocd_60p_60n_diff (I/O), lpddr4_odt_60_diff (Input), lpddr4_ocd_80p_80n_diff (I/O), lpddr4_ocd_120pd_60p_40n_diff (I/O), lpddr4_odt_80_diff (Input), lpddr4_odt_off_diff (Input), lpddr4_ocd_120pd_48p_40n (I/O), lpddr4_ocd_120pd_48p_40n_diff (I/O), ddr4_ocd_34p_34n (I/O), ddr4_ocd_40p_40n (I/O), ddr4_ocd_48p_48n (I/O), ddr4_ocd_60p_60n (I/O), ddr4_ocd_80p_80n (I/O), ddr4_ocd_34p_34n_diff (I/O), ddr4_ocd_40p_40n_diff (I/O), ddr4_ocd_48p_48n_diff (I/O), ddr4_ocd_60p_60n_diff (I/O), ddr4_ocd_80p_80n_diff (I/O), ddr4_odt_34 (Input), ddr4_odt_40 (Input), ddr4_odt_48 (Input), ddr4_odt_60 (Input), ddr4_odt_80 (Input), ddr4_odt_120 (Input), ddr4_odt_240 (Input), ddr4_odt_off (Input), ddr4_odt_34_diff (Input), ddr4_odt_40_diff (Input), ddr4_odt_48_diff (Input), ddr4_odt_60_diff (Input), ddr4_odt_80_diff (Input), ddr4_odt_120_diff (Input), ddr4_odt_240_diff (Input), ddr4_odt_off_diff (Input), lp4x_ocd_40p_40n (I/O), lp4x_ocd_120p_120n (I/O), lp4x_ocd_48p_48n (I/O), lp4x_ocd_34p_34n (I/O), lp4x_ocd_80p_80n (I/O), lp4x_ocd_240p_240n (I/O), lp4x_ocd_60p_60n (I/O), lp4x_0p6_ocd_80p_80n (I/O), lp4x_0p6_ocd_40p_40n (I/O), lp4x_odt_120 (Input), lp4x_odt_40 (Input), lp4x_odt_48 (Input), lp4x_odt_60 (Input), lp4x_odt_80 (Input), lp4x_odt_off (Input), lp4x_ocd_40p_40n_diff (I/O)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
